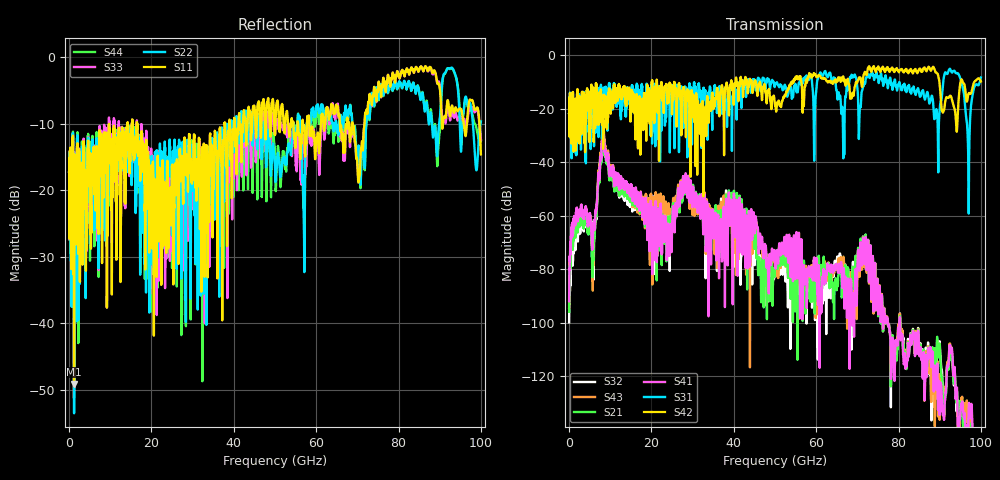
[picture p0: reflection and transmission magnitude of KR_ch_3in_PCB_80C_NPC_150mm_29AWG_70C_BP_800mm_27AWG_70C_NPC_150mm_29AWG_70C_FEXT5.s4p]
# GHz S RI R 45
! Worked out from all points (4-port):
!   4000 points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, 25 MHz to 100 GHz, reference 45 ohm
!   strongest paths, dB at 25 MHz, 25.02 GHz, 50.02 GHz, 75.03 GHz, 100 GHz:
!     S42: -21.8, -20.6, -18.8, -4.2, -9.7
!     S31: -21.8, -12.0, -11.2, -8.1, -8.3
!     S41: -92.0, -62.6, -76.5, -94.2, -155.4
!     S21: -96.0, -58.8, -78.9, -94.7, -167.9
!     S43: -94.5, -59.7, -79.4, -94.1, -166.5
!     S32: -100.0, -63.3, -82.4, -94.7, -171.7
!   lowest |S11| = -49.1 dB at 1.225 GHz (marker M1), VSWR 1.01, Z = 45.3 - j0.0216 ohm
!   |S11| at or under -10 dB: start of sweep to 14.15 GHz; 16.48 GHz to 37.76 GHz (21.28 GHz wide, 78.5 % of centre); 68.84 GHz to 71.75 GHz (2.903 GHz wide, 4.13 % of centre)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
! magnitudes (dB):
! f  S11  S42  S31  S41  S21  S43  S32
! 25 MHz  -17.2  -21.8  -21.8  -92.0  -96.0  -94.5  -100.0
! 1.225 GHz  -49.1  -27.8  -27.2  -61.2  -65.0  -63.4  -68.3
! 5.95 GHz  -16.5  -14.1  -14.7  -63.2  -73.3  -72.3  -74.2
! 8.375 GHz  -20.9  -22.3  -19.2  -29.1  -30.6  -27.3  -28.8
! 24.07 GHz  -23.5  -15.7  -15.3  -63.9  -61.8  -55.6  -59.1
! 96.92 GHz  -7.7  -14.7  -36.8  -138.8  -142.4  -140.9  -146.8
! 100 GHz  -14.6  -9.7  -8.3  -155.4  -167.9  -166.5  -171.7
